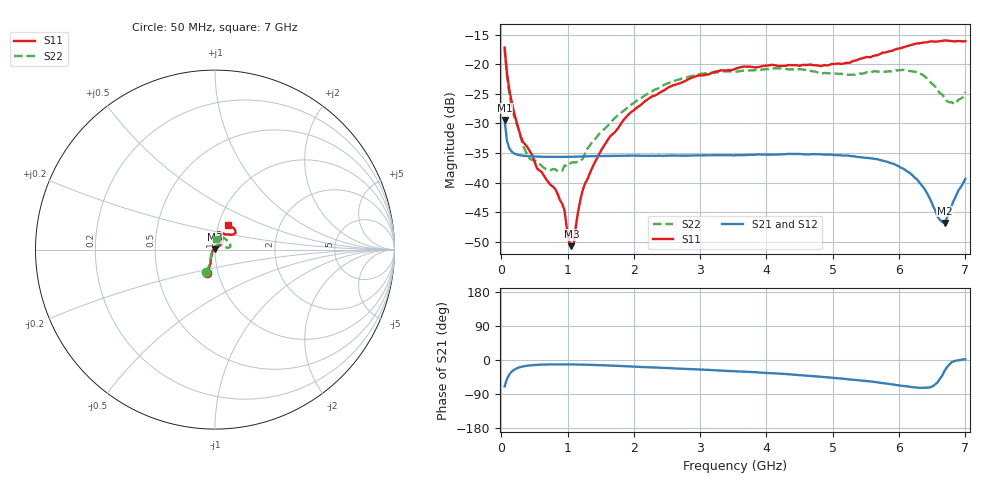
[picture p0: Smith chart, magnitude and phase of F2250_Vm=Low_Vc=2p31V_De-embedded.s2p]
! Integrated Device Technology
! Corporate Headquarters
! 6024 Silver Creek Valley Road
! San Jose, CA 95138  USA
! Phone:  1-408-284-8200
! Toll Free:  1-800-223-1366
! Webpage:  http://www.idt.com/
! Timing and RF Division
! 515 Groton Road, Suite 102
! Westford, MA 01886-6024
! Device:  F2250
! Description: Voltage Variable RF Attenuator
! Frequency:  50.0 -  6000.00 MHz
! Package:  3x3 mm Thin QFN Plastic Package: 16 pin
! Ports:  2 RF, 3 DC
!  Pin  1  = GND
!  Pin  2  = NC
!  Pin  3  = RF1  = Port 1
!  Pin  4  = NC
!  Pin  5  = GND
!  Pin  6  = GND
!  Pin  7  = GND
!  Pin  8  = GND
!  Pin  9  = NC
!  Pin 10  = RF2  = Port 2
!  Pin 11  = NC
!  Pin 12  = GND
!  Pin 13  = GND
!  Pin 14  = VCNTRL
!  Pin 15  = VDD
!  Pin 16  = VMODE
! Vcntrl:  2.310 Volts
! Vmode:  +0.000 Volts
! Vdd:  +3.30  Volts
! Current:  1.176 mA
! Data:  The device was measured on a the F2250 evaluation board which has
!  individual transmission lines to the RF pins.  Data was collected
!  using a calibrated network analyzer.  The evaluation board was
!  de-embedded using a TRL calibration technique.
!  The reference plane is the edge of the package pin.
! Misc:  SN 10
!  Action Tracker AT0258
! Date Measured:  2014-11-26
! Date:  2015-10-15  MJV
! Note:
!  Integrated Device Technology supplies this data as a sample of measured
!  data at the package pin for this product.  Your particular data for this
!  product may vary.
!  Data was taken at 25 degrees C.
!  Integrated Device Technology reserves the right to change this data at anytime.
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# GHz S dB R 50
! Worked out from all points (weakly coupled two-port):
!   201 points, 50 MHz to 7 GHz, reference 50 ohm
!   highest |S21| = -29.40 dB at 50 MHz (marker M1); lowest = -46.8 dB at 6.687 GHz (marker M2)
!   lowest |S11| = -50.7 dB at 1.058 GHz (marker M3), VSWR 1.01, Z = 49.8 + j0.242 ohm
!   |S11| at or under -10 dB: start of sweep to end of sweep
!   |S22| runs from -38.1 to -17.3 dB; largest |S21 - S12| = 6.7e-05
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0.05  -17.18 -108.6  -29.40 -69.7  -29.40 -69.7  -17.31 -110.8
0.08475  -21.44 -107.5  -32.90 -50.2  -32.90 -50.3  -21.81 -109.8
0.15425  -26.23 -116.6  -34.73 -31.1  -34.73 -31.1  -26.93 -121.5
0.29325  -32.20 -127.7  -35.40 -18.4  -35.40 -18.4  -32.34 -136.2
0.3975  -34.08 -141.7  -35.53 -15.0  -35.53 -15.0  -35.45 -159.5
0.5365  -37.56 -155.6  -35.60 -12.8  -35.61 -12.8  -36.52 178.3
0.91875  -43.57 158.0  -35.66 -11.5  -35.65 -11.5  -37.98 131.4
0.9535  -44.67 169.9  -35.65 -11.5  -35.66 -11.5  -37.09 129.3
1.023  -49.96 144.2  -35.65 -11.6  -35.64 -11.6  -36.93 113.4
1.05775  -50.73 123.2  -35.64 -11.6  -35.64 -11.6  -36.59 108.3
1.0925  -50.37 89.9  -35.63 -11.7  -35.63 -11.7  -36.57 103.4
1.162  -44.65 56.7  -35.61 -11.9  -35.61 -11.9  -36.44 92.5
1.2315  -41.12 44.4  -35.58 -12.1  -35.58 -12.1  -35.91 83.1
1.6485  -32.11 42.0  -35.49 -14.7  -35.49 -14.7  -29.88 63.2
2.37825  -24.87 47.4  -35.45 -20.3  -35.45 -20.3  -24.01 56.1
3.525  -20.80 72.5  -35.38 -29.6  -35.38 -29.6  -21.26 74.5
4.7065  -20.17 72.4  -35.18 -42.6  -35.18 -42.6  -21.22 72.1
5.85325  -17.82 40.5  -36.61 -63.3  -36.61 -63.3  -21.17 22.6
6.27025  -16.50 40.1  -39.46 -72.6  -39.46 -72.7  -21.39 9.2
6.68725  -15.99 48.8  -46.80 -28.3  -46.78 -27.9  -25.72 28.1
6.861  -16.13 55.1  -42.17 -1.7  -42.13 -1.6  -26.56 57.9
7  -16.12 63.3  -39.35 1.6  -39.30 1.5  -24.70 83.3
